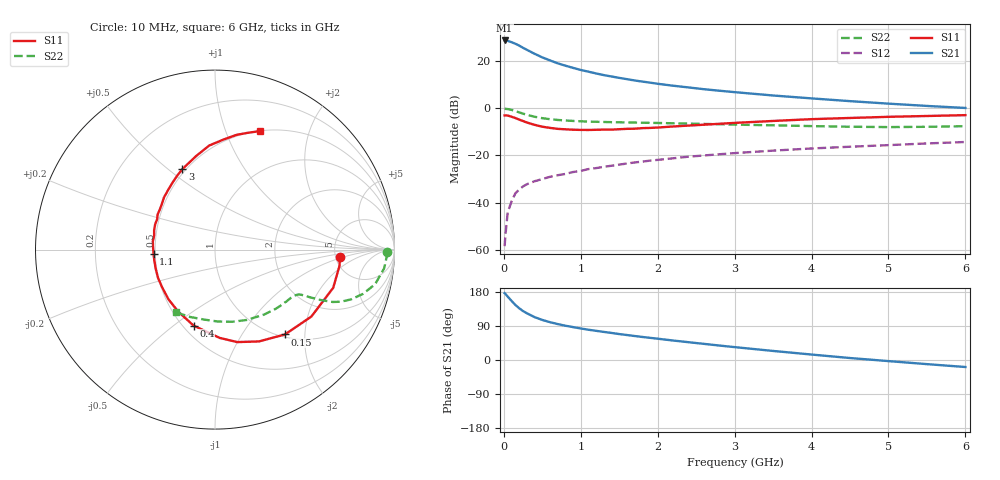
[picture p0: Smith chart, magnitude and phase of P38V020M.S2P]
! SIEMENS Small Signal Semiconductors
! BFP181
! Si NPN RF Bipolar Junction Transistor in SOT143
! VCE = 8 V  IC = 20 mA
! Common Emitter S-Parameters:  March  1996
# GHz  S  MA  R  50
!  f  S11  S21  S12  S22
! GHz  MAG  ANG  MAG  ANG  MAG  ANG  MAG  ANG
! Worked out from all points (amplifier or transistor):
!   36 points, 10 MHz to 6 GHz, reference 50 ohm
!   highest |S21| = 28.5 dB at 10 MHz (marker M1)
!   |S21| within 3 dB of that: start of sweep to 243.4 MHz
!   unconditionally stable (mu >= 1): 887.8 MHz to end of sweep
!   at 250 MHz: K = 0.45, MSG = 29.3 dB, |S12| = -33.2 dB
!   at 1.4 GHz: K = 1.15, MAG = 16.5 dB, |S12| = -24.4 dB
!   at 6 GHz: K = 1.02, MAG = 6.4 dB, |S12| = -14.4 dB
!   S11 on the Smith chart (normalised r, x): 10 MHz: 5.48, -0.83; 150 MHz: 1.05, -1.59; 400 MHz: 0.56, -0.59; 1.1 GHz: 0.49, -0.02; 3 GHz: 0.48, +0.56; 6 GHz: 0.50, +1.32
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0.01  0.6972 -3.2  26.74 176.4  0.0012 77.4  0.9598 -0.8
0.02  0.6997 -7.3  26.65 174.7  0.002 76.1  0.958 -2.2
0.05  0.6922 -17.9  26.25 167.4  0.0062 81.4  0.9483 -6.3
0.1  0.6537 -34.8  24.58 156.0  0.0106 73.3  0.9129 -12.2
0.15  0.6127 -50.5  22.79 145.3  0.0157 66.1  0.8599 -16.7
0.2  0.5673 -64.4  20.8 136.5  0.019 62.9  0.8071 -20.1
0.25  0.5299 -76.5  18.66 129.1  0.022 60.0  0.7591 -22.5
0.3  0.4926 -87.0  16.94 123.3  0.0245 57.1  0.7173 -24.0
0.4  0.4397 -105.8  13.97 113.1  0.0283 54.8  0.6524 -25.5
0.5  0.4021 -120.5  11.72 105.7  0.0315 53.7  0.6092 -26.3
0.6  0.3795 -133.0  10.14 99.8  0.0351 53.4  0.5795 -26.9
0.7  0.362 -144.3  8.786 94.8  0.0379 53.5  0.5584 -27.2
0.9  0.3474 -161.7  7.046 86.8  0.0443 54.4  0.5322 -28.0
1.1  0.3432 -176.3  5.851 79.9  0.0512 54.5  0.516 -29.5
1.3  0.3492 172.5  4.952 74.1  0.0571 54.1  0.5061 -31.5
1.6  0.3623 156.9  4.063 65.9  0.0671 53.3  0.4947 -34.7
2.2  0.4065 134.4  2.956 51.4  0.0864 50.4  0.4751 -43.0
3  0.4838 112.1  2.161 34.0  0.1112 44.4  0.4454 -56.2
3.5  0.5317 101.4  1.836 23.9  0.1255 40.5  0.4301 -65.7
4.5  0.6149 85.6  1.395 5.2  0.1517 32.1  0.4014 -87.4
5.5  0.6771 74.1  1.105 -10.9  0.178 24.8  0.4001 -110.4
6  0.7056 69.3  1.001 -18.5  0.191 20.5  0.4118 -122.0
